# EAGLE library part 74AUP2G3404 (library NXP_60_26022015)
Short Description AAL Eindhoven MK
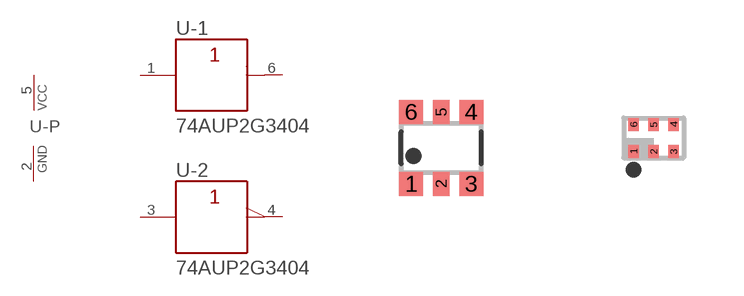
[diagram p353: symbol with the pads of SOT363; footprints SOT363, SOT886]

Designator prefix U; gates -1=BUFFER -2=INVERTER -P=PWRN

## 74AUP2G3404GW  [SOT363]
1  -1:A  in
2  -P:GND  pwr
3  -2:A  in
4  -2:Y  out
5  -P:VCC  pwr
6  -1:Y  out

## 74AUP2G3404GM  [SOT886]
Pads as for SOT363

## 74AUP2G3404GF  [SOT891]
Pads as for SOT363

## 74AUP2G3404GN  [SOT1115]
Pads as for SOT363

## 74AUP2G3404GS  [SOT1202]
Pads as for SOT363

## Footprint SOT363 (pad centres in mm)
SOT363 Plastic surface-mounted package; 6 leads JEDEC: -- IEC: -- JEITA: SC-88
smd 0.6 x 0.6: 1 -0.75,-0.9; 3 0.75,-0.9; 4 0.75,0.9; 6 -0.75,0.9
smd 0.4 x 0.6: 2 0,-0.9; 5 0,0.9

## Footprint SOT886 (pad centres in mm)
SOT886 XSON6: plastic extremely thin small outline package; no leads; 6 terminals; body 1 x 1.45 x 0.5 mm JEDEC: MO-252 IEC: ---
smd 0.27 x 0.325: 1 -0.5,-0.338; 2 0,-0.338; 3 0.5,-0.338; 4 0.5,0.338; 5 0,0.338; 6 -0.5,0.338

## Footprint SOT891 (pad centres in mm)
SOT891 XSON6: plastic extremely thin small outline package; no leads; 6 terminals; body 1 x 1 x 0.5 mm JEDEC: -- IEC: ---
smd 0.15 x 0.5: 1 -0.35,-0.35; 2 0,-0.35; 3 0.35,-0.35; 4 0.35,0.35; 5 0,0.35; 6 -0.35,0.35

## Footprint SOT1115 (pad centres in mm)
!!!!!!Experimental, not tested!!!!!!!!!!!! MK SOT1115 XSON6: extremely thin small outline package; no leads; 6 terminals; body 0.9 x 1.0 x 0.35 mm JEDEC: -- IEC: -- JEITA: --
smd 0.22 x 0.325: 1 -0.3,-0.312; 2 0,-0.312; 3 0.3,-0.312; 4 0.3,0.312; 5 0,0.312; 6 -0.3,0.312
